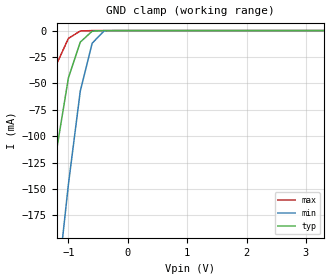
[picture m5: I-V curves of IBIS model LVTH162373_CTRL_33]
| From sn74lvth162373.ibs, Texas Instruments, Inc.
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|   Model LVTH162373 Input_CTRL_33
[Model]   LVTH162373_CTRL_33
Model_type  Input
Polarity   Inverting
Vinl = 0.8V
Vinh = 2.0V
| variable   typ   min   max
C_comp   3p   NA   NA
[Temperature Range]   25   -40   85
[Voltage range]   3.3   3.0   3.6
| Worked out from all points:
|   GND clamp passes 1 mA (typ) near -0.61 V on its own axis
|Process range|   weak   strong
[GND Clamp]
|   25C:3.3V   -40C:3.0V   85C:3.6V
|   Voltage   I(typ)   I(min)   I(max)
-5V       -1.927A    -2.225A    -1.638A
-1.8V     -399.9mA   -561.6mA   -252.6mA
-1.6V     -304.4mA   -457.6mA   -166mA
-1.4V     -209mA     -353.6mA   -82.92mA
-1.2V     -113.6mA   -249.7mA   -31.94mA
-1V       -44.85mA   -145.7mA   -7.401mA
-800mV    -10.91mA   -57.38mA   -419.1uA
-600mV    -585.2uA   -11.98mA   -1.324uA
-400mV    -1.195uA   -364.3uA   -1.888nA
3.3V      -82.78pA   93.68nA    -108.8pA
